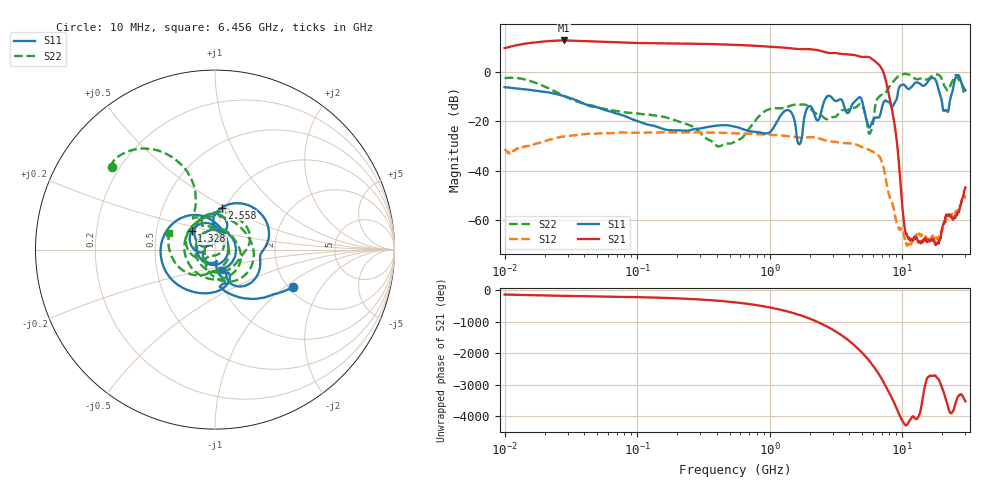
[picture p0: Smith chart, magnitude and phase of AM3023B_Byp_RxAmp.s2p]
# Hz S DB R 50.0
!freq dBS11 angS11 dBS21 angS21 dBS12 angS12 dBS22 angS22
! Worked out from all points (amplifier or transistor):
!   1601 points, 10 MHz to 30 GHz, reference 50 ohm
!   highest |S21| = 12.5 dB at 28.17 MHz (marker M1)
!   |S21| within 3 dB of that: 10.17 MHz to 1.346 GHz (1.336 GHz wide, 197 % of centre)
!   unconditionally stable (mu >= 1): start of sweep to end of sweep
!   at 37.85 MHz: K = 2.17, MAG = 12.7 dB, |S12| = -25.4 dB
!   at 547.7 MHz: K = 2.62, MAG = 10.8 dB, |S12| = -24.9 dB
!   at 30 GHz: K = 24187.86, MAG = -45.3 dB, |S12| = -49.8 dB
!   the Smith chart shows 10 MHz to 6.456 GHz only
!   S11 on the Smith chart (normalised r, x): 10 MHz: 2.12, -1.15; 1.328 GHz: 0.76, +0.16; 2.558 GHz: 0.96, +0.48; 6.456 GHz: 1.06, -0.24
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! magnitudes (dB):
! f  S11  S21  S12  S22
! 10 MHz  -6.3  9.4  -31.3  -2.7
! 28.17 MHz  -9.9  12.5  -26.2  -9.9
! 38.04 MHz  -12.5  12.3  -25.4  -12.7
! 144.7 MHz  -22.4  11.4  -24.6  -17.9
! 547.7 MHz  -22.3  10.7  -24.9  -28.2
! 969 MHz  -24.8  10.1  -25.4  -15.4
! 1.328 GHz  -15.7  9.5  -25.9  -14.4
! 1.68 GHz  -29.3  9.0  -26.6  -13.3
! 2.084 GHz  -14.6  8.9  -26.5  -15.5
! 2.314 GHz  -19.7  8.6  -26.8  -17.1
! 2.558 GHz  -12.5  8.0  -27.6  -18.5
! 4.854 GHz  -10.5  6.0  -30.2  -13.0
! 5.725 GHz  -22.1  5.6  -31.7  -24.9
! 6.456 GHz  -18.5  3.4  -33.3  -11.3
! 7.926 GHz  -12.3  -9.1  -49.3  -6.6
! 9.027 GHz  -11.5  -26.3  -60.2  -2.6
! 10.33 GHz  -5.3  -61.1  -65.6  -1.0
! 11.19 GHz  -7.1  -67.1  -69.5  -1.2
! 18.37 GHz  -5.1  -69.3  -67.1  -1.2
! 21.35 GHz  -15.5  -58.3  -60.5  -6.8
! 25.82 GHz  -1.7  -57.8  -56.3  -1.5
! 30 GHz  -7.6  -46.7  -49.8  -9.3
